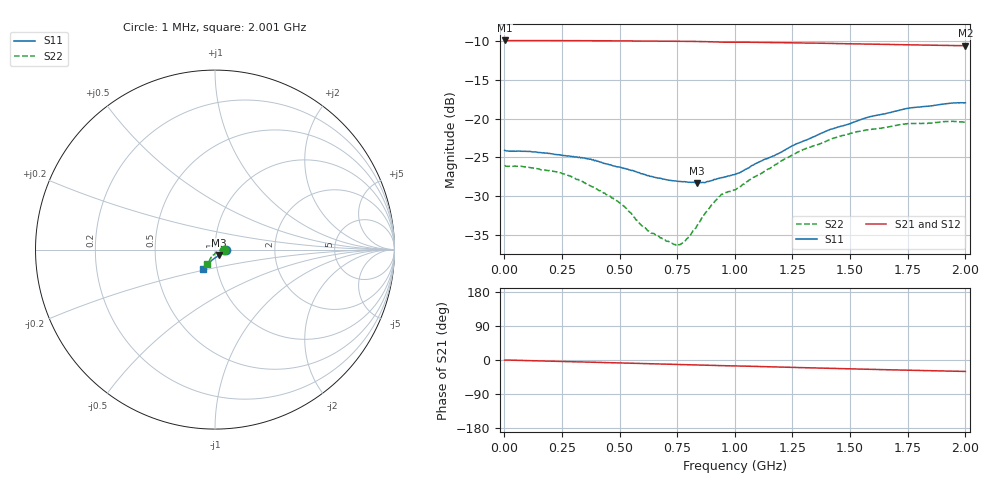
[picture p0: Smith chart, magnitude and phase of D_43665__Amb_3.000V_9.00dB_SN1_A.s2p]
! device id: 43665_
! dir: \\malibu\benchdata\1_engineers\tn_data\43665_75ohm\new\sparar\43665_\amb\3p000v\9p00db
! Serial: 1
! Insertion: A
! Temp: Amb
! VDD: 3.000V
! Attenuation Step: 9.00dB
! IDD: 1.453127e+00mA
! FILE NAME
! DATE 03-27-2009 08:35:34
! CORRECTED  DATA
#  Hz  S  RI  R  75
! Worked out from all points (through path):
!   401 points, 1 MHz to 2.001 GHz, reference 75 ohm
!   highest |S21| = -9.97 dB at 1 MHz (marker M1); lowest = -10.6 dB at 2.001 GHz (marker M2)
!   group delay of S21, straight-line fit = 42.7 ps
!   lowest |S11| = -28.3 dB at 836 MHz (marker M3), VSWR 1.08, Z = 77.9 - j5.12 ohm
!   |S11| at or under -10 dB: start of sweep to end of sweep
!   |S22| runs from -36.4 to -20.3 dB; largest |S21 - S12| = 0.0012
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1000000  0.0625 -0.000777  0.3172 -0.000606  0.3173 -0.000514  0.05 -0.000329
2.21e8  0.0586 -0.00543  0.3159 -0.0185  0.316 -0.0185  0.0455 0.00197
3.36e8  0.0554 -0.00948  0.3148 -0.0282  0.3149 -0.0283  0.0394 0.00295
4.96e8  0.0465 -0.0152  0.3126 -0.0419  0.3127 -0.0419  0.0291 -0.00109
5.41e8  0.0436 -0.0171  0.3116 -0.0457  0.3117 -0.0457  0.0251 -0.00253
5.96e8  0.0396 -0.0196  0.3105 -0.0502  0.3105 -0.0502  0.0201 -0.00416
6.71e8  0.0341 -0.0236  0.309 -0.0565  0.309 -0.0566  0.0152 -0.00864
7.41e8  0.0285 -0.0276  0.3073 -0.0627  0.3074 -0.0626  0.00995 -0.012
7.56e8  0.0274 -0.0285  0.3069 -0.064  0.3069 -0.0639  0.00831 -0.0131
7.96e8  0.024 -0.0308  0.3057 -0.0675  0.3057 -0.0675  0.00475 -0.0164
8.36e8  0.0204 -0.0328  0.3044 -0.071  0.3043 -0.0709  0.00131 -0.0205
8.76e8  0.0162 -0.0357  0.3026 -0.0747  0.3027 -0.0744  -0.00161 -0.0251
9.31e8  0.0105 -0.04  0.2996 -0.0788  0.2998 -0.0785  -0.00882 -0.0302
9.51e8  0.00883 -0.041  0.2988 -0.0798  0.2989 -0.0795  -0.0123 -0.0307
1.001e9  0.00418 -0.0436  0.2978 -0.0827  0.298 -0.0825  -0.0166 -0.0307
1.211e9  -0.0177 -0.0596  0.2905 -0.0996  0.291 -0.0995  -0.0247 -0.0484
1.336e9  -0.0296 -0.0697  0.285 -0.1084  0.2855 -0.1084  -0.0306 -0.0589
1.406e9  -0.0364 -0.0759  0.2818 -0.1138  0.2824 -0.114  -0.0314 -0.0655
1.521e9  -0.0462 -0.0835  0.2763 -0.1209  0.2768 -0.1212  -0.0377 -0.0723
1.671e9  -0.0566 -0.0933  0.2692 -0.1302  0.2693 -0.1307  -0.0411 -0.0785
1.766e9  -0.0618 -0.0997  0.2646 -0.1356  0.2648 -0.1365  -0.0422 -0.0829
2.001e9  -0.0686 -0.106  0.2537 -0.1476  0.2529 -0.1485  -0.0465 -0.0823
